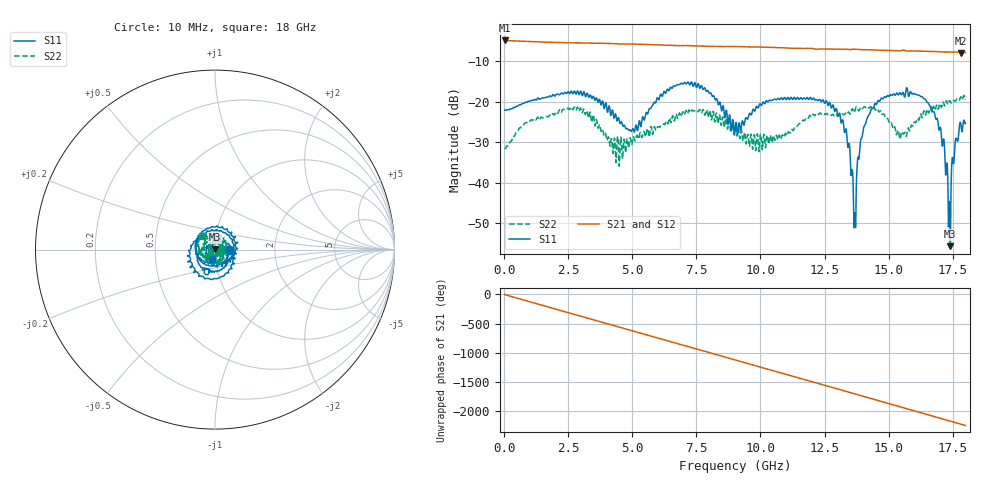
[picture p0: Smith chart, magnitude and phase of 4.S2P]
!Agilent Technologies,E5071C,MY46316741,A.11.02
!Date: Fri May 06 15:19:20 2022
!Data & Calibration Information:
!Freq	S11:SOLT2(ON)	S21:SOLT2(ON)	S12:SOLT2(ON)	S22:SOLT2(ON)
!PortZ  Port1:50+j0  Port2:50+j0
!Above PortZ is port z conversion or system Z0 setting when saving the data.
!When reading, reference impedance value at option line is always used.
# Hz S dB R 50
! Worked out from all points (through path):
!   1800 points, 10 MHz to 18 GHz, reference 50 ohm
!   highest |S21| = -4.94 dB at 10 MHz (marker M1); lowest = -8.0 dB at 17.84 GHz (marker M2)
!   group delay of S21, straight-line fit = 347 ps
!   lowest |S11| = -55.6 dB at 17.41 GHz (marker M3), VSWR 1.00, Z = 50 + j0.163 ohm
!   |S11| at or under -10 dB: start of sweep to end of sweep
!   |S22| runs from -36.0 to -18.5 dB; largest |S21 - S12| = 0.034
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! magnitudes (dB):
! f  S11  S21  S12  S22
! 10 MHz  -22.1  -4.9  -5.0  -31.4
! 3.01 GHz  -17.9  -5.5  -5.6  -22.3
! 4.42 GHz  -24.5  -5.8  -5.8  -28.6
! 5 GHz  -26.8  -5.8  -5.8  -29.8
! 6.01 GHz  -19.4  -6.0  -6.0  -26.2
! 7.5 GHz  -16.5  -6.3  -6.3  -22.1
! 9.01 GHz  -26.6  -6.5  -6.5  -26.3
! 10.01 GHz  -20.8  -6.6  -6.6  -28.1
! 12.01 GHz  -19.5  -6.9  -7.0  -23.5
! 13.15 GHz  -25.2  -7.1  -7.1  -23.3
! 13.41 GHz  -31.3  -7.1  -7.2  -22.8
! 13.67 GHz  -47.5  -7.1  -7.1  -22.5
! 13.86 GHz  -33.0  -7.2  -7.4  -22.2
! 14.1 GHz  -25.5  -7.2  -7.3  -21.5
! 15.01 GHz  -18.7  -7.4  -7.4  -24.9
! 15.64 GHz  -18.8  -7.4  -7.8  -27.6
! 16.71 GHz  -22.2  -7.7  -7.7  -22.2
! 17.1 GHz  -31.0  -7.8  -7.8  -20.6
! 17.41 GHz  -55.6  -7.8  -7.9  -20.0
! 17.55 GHz  -35.0  -7.8  -7.9  -19.8
! 17.84 GHz  -26.5  -8.0  -8.0  -19.0
! 18 GHz  -25.4  -7.9  -8.1  -19.6
